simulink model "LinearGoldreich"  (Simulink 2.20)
settings: Solver=ode45  StartTime=0.0  StopTime=2  RelTol=1e-3  AbsTol=1e-6
libraries: simulink x1

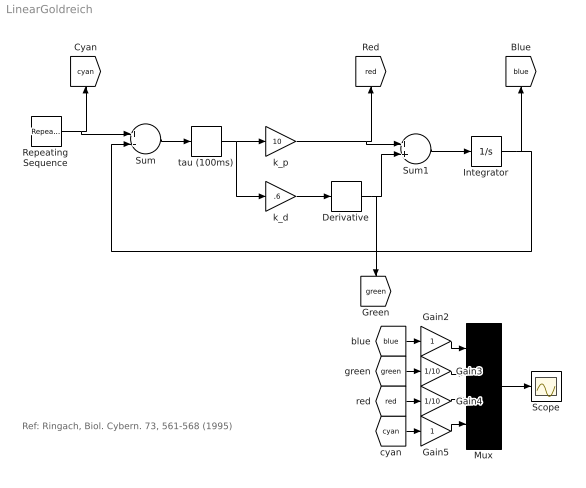
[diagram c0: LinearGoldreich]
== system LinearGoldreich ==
  note: Ref: Ringach, Biol. Cybern. 73, 561-568 (1995)
  Derivative : Derivative
  Gain2 : Gain  Gain=1
  Gain3 : Gain  Gain=1/10
  Gain4 : Gain  Gain=1/10
  Gain5 : Gain  Gain=1
  Integrator : Integrator  ExternalReset=none  InitialConditionSource=internal  InitialCondition=0  LimitOutput=off  UpperSaturationLimit=inf  LowerSaturationLimit=-inf  ShowSaturationPort=off  ShowStatePort=off  AbsoluteTolerance=auto
  Mux : Mux  Inputs=4
  Repeating Sequence : simulink/Sources/Repeating Sequence  rep_seq_t=[0 .1 .10001 3 3.0001 6]  rep_seq_y=[0 0 20 20 0 0]
  Scope : Scope
  Sum : Sum  Inputs=+-
  Sum1 : Sum  Inputs=++
  k_d : Gain  Gain=.6
  k_p : Gain  Gain=10
  tau (100ms) : TransportDelay  DelayTime=80e-3  InitialInput=0  BufferSize=1024
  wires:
  Sum/1 -> tau (100ms)/1
  Repeating Sequence/1 -> Sum/1, [cyan]
  Mux/1 -> Scope/1
  [blue] -> Gain2/1
  Gain2/1 -> Mux/1
  [green] -> Gain3/1
  Gain3/1 -> Mux/2
  [red] -> Gain4/1
  Gain4/1 -> Mux/3
  [cyan] -> Gain5/1
  Gain5/1 -> Mux/4
  tau (100ms)/1 -> k_p/1, k_d/1
  k_d/1 -> Derivative/1
  Sum1/1 -> Integrator/1
  Integrator/1 -> Sum/2, [blue]
  Derivative/1 -> Sum1/2, [green]
  k_p/1 -> Sum1/1, [red]
